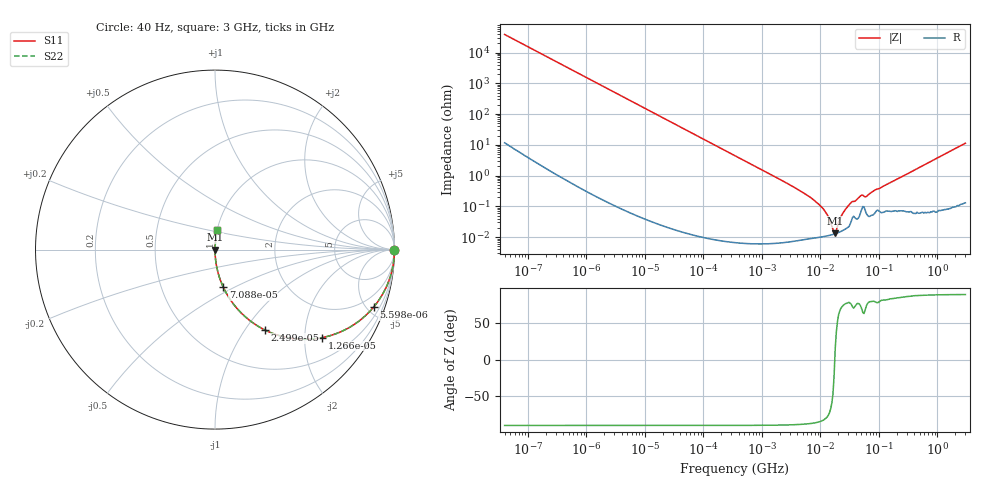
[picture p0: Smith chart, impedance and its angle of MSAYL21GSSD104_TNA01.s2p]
! MSAYL21GSSD104_TNA01  S-PARAMETER MODEL  ( General Type )
! Model Generated by TAIYO YUDEN Corporation (http://www.ty-top.com)
! Version 2.0
! TAIYO YUDEN Control No. 031016
! Copyright(c) 2003 TAIYO YUDEN CO.,LTD. All Rights Reserved.
! Product Description (link to TY-COMPAS)
! https://ds.yuden.co.jp/TYCOMPAS/or/detail?pn=MSAYL21GSSD104KTNA01&u=M
! Products Name : Multilayer Ceramic Capacitors
! Characteristics :
!  Capacitance : 0.1 uF , Rated Voltage : 10V
!  Case Size : 2.0 x 1.25 / 0.079 x 0.049 [mm/inch] , Thickness : 1.25 / 0.049 [mm/inch]
!  (Conditions: Temperature = 25 degC , DC Bias Current/Voltage = 0A / 0V)
! External Node Assignments :
!  1  o---| |---o  2
! GND o---------o GND
! Frequency Range : 40Hz  -  3GHz  [ 401 STEP ]
# MHz S RI R 50
! Freq[MHz].  S11 Real  S11 Imag  S21 Real  S21 Imag  S12 Real  S12 Imag  S22 Real  S22 Imag
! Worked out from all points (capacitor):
!   401 points, 40 Hz to 3 GHz, reference 50 ohm
!   read as one part in series: C = 103 nF near 44 Hz
!   lowest |Z| = 13.4 mohm at 17.88 MHz (marker M1)
!   series resonance near 17.56 MHz, so ESL is about 800 pH
!   S11 on the Smith chart (normalised r, x): 40 Hz: open; 5.598 kHz: 1.00, -5.51; 12.66 kHz: 1.00, -2.44; 24.99 kHz: 1.00, -1.23; 70.88 kHz: 1.00, -0.44; 3 GHz: 1.00, +0.23
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4e-05  1 -0.00259  7.51e-06 0.00259  7.51e-06 0.00259  1 -0.00259
0.000834  0.9971 -0.0539  0.00293 0.0539  0.00293 0.0539  0.9971 -0.0539
0.002366  0.977 -0.1499  0.023 0.1499  0.023 0.1499  0.977 -0.1499
0.005598  0.8835 -0.3207  0.1165 0.3207  0.1165 0.3207  0.8835 -0.3207
0.012659  0.5975 -0.4903  0.4025 0.4903  0.4025 0.4903  0.5975 -0.4903
0.017386  0.4404 -0.4963  0.5596 0.4963  0.5596 0.4963  0.4404 -0.4963
0.024987  0.276 -0.4468  0.724 0.4468  0.724 0.4468  0.276 -0.4468
0.041141  0.1233 -0.3286  0.8767 0.3286  0.8767 0.3286  0.1233 -0.3286
0.07088  0.0453 -0.2077  0.9547 0.2077  0.9547 0.2077  0.0453 -0.2077
0.362475  0.00187 -0.0425  0.9981 0.0425  0.9981 0.0425  0.00187 -0.0425
2.916825  9.61e-05 -0.00514  0.9999 0.00514  0.9999 0.00514  9.61e-05 -0.00514
7.222098  9.41e-05 -0.00177  0.9999 0.00177  0.9999 0.00177  9.41e-05 -0.00177
11.89125  0.000106 -0.000691  0.9999 0.000691  0.9999 0.000691  0.000106 -0.000691
13.62356  0.000112 -0.000448  0.9999 0.000448  0.9999 0.000448  0.000112 -0.000448
16.33207  0.000122 -0.000134  0.9999 0.000134  0.9999 0.000134  0.000122 -0.000134
17.88201  0.000129 3.54e-05  0.9999 -3.54e-05  0.9999 -3.54e-05  0.000129 3.54e-05
23.47158  0.00016 0.000517  0.9998 -0.000517  0.9998 -0.000517  0.00016 0.000517
32.2371  0.00027 0.00121  0.9997 -0.00121  0.9997 -0.00121  0.00027 0.00121
48.47801  0.000624 0.00211  0.9994 -0.00211  0.9994 -0.00211  0.000624 0.00211
60.81113  0.00059 0.00201  0.9994 -0.00201  0.9994 -0.00201  0.00059 0.00201
150.5692  0.000723 0.00564  0.9993 -0.00564  0.9993 -0.00564  0.000723 0.00564
3000  0.0138 0.1111  0.9862 -0.1111  0.9862 -0.1111  0.0138 0.1111
